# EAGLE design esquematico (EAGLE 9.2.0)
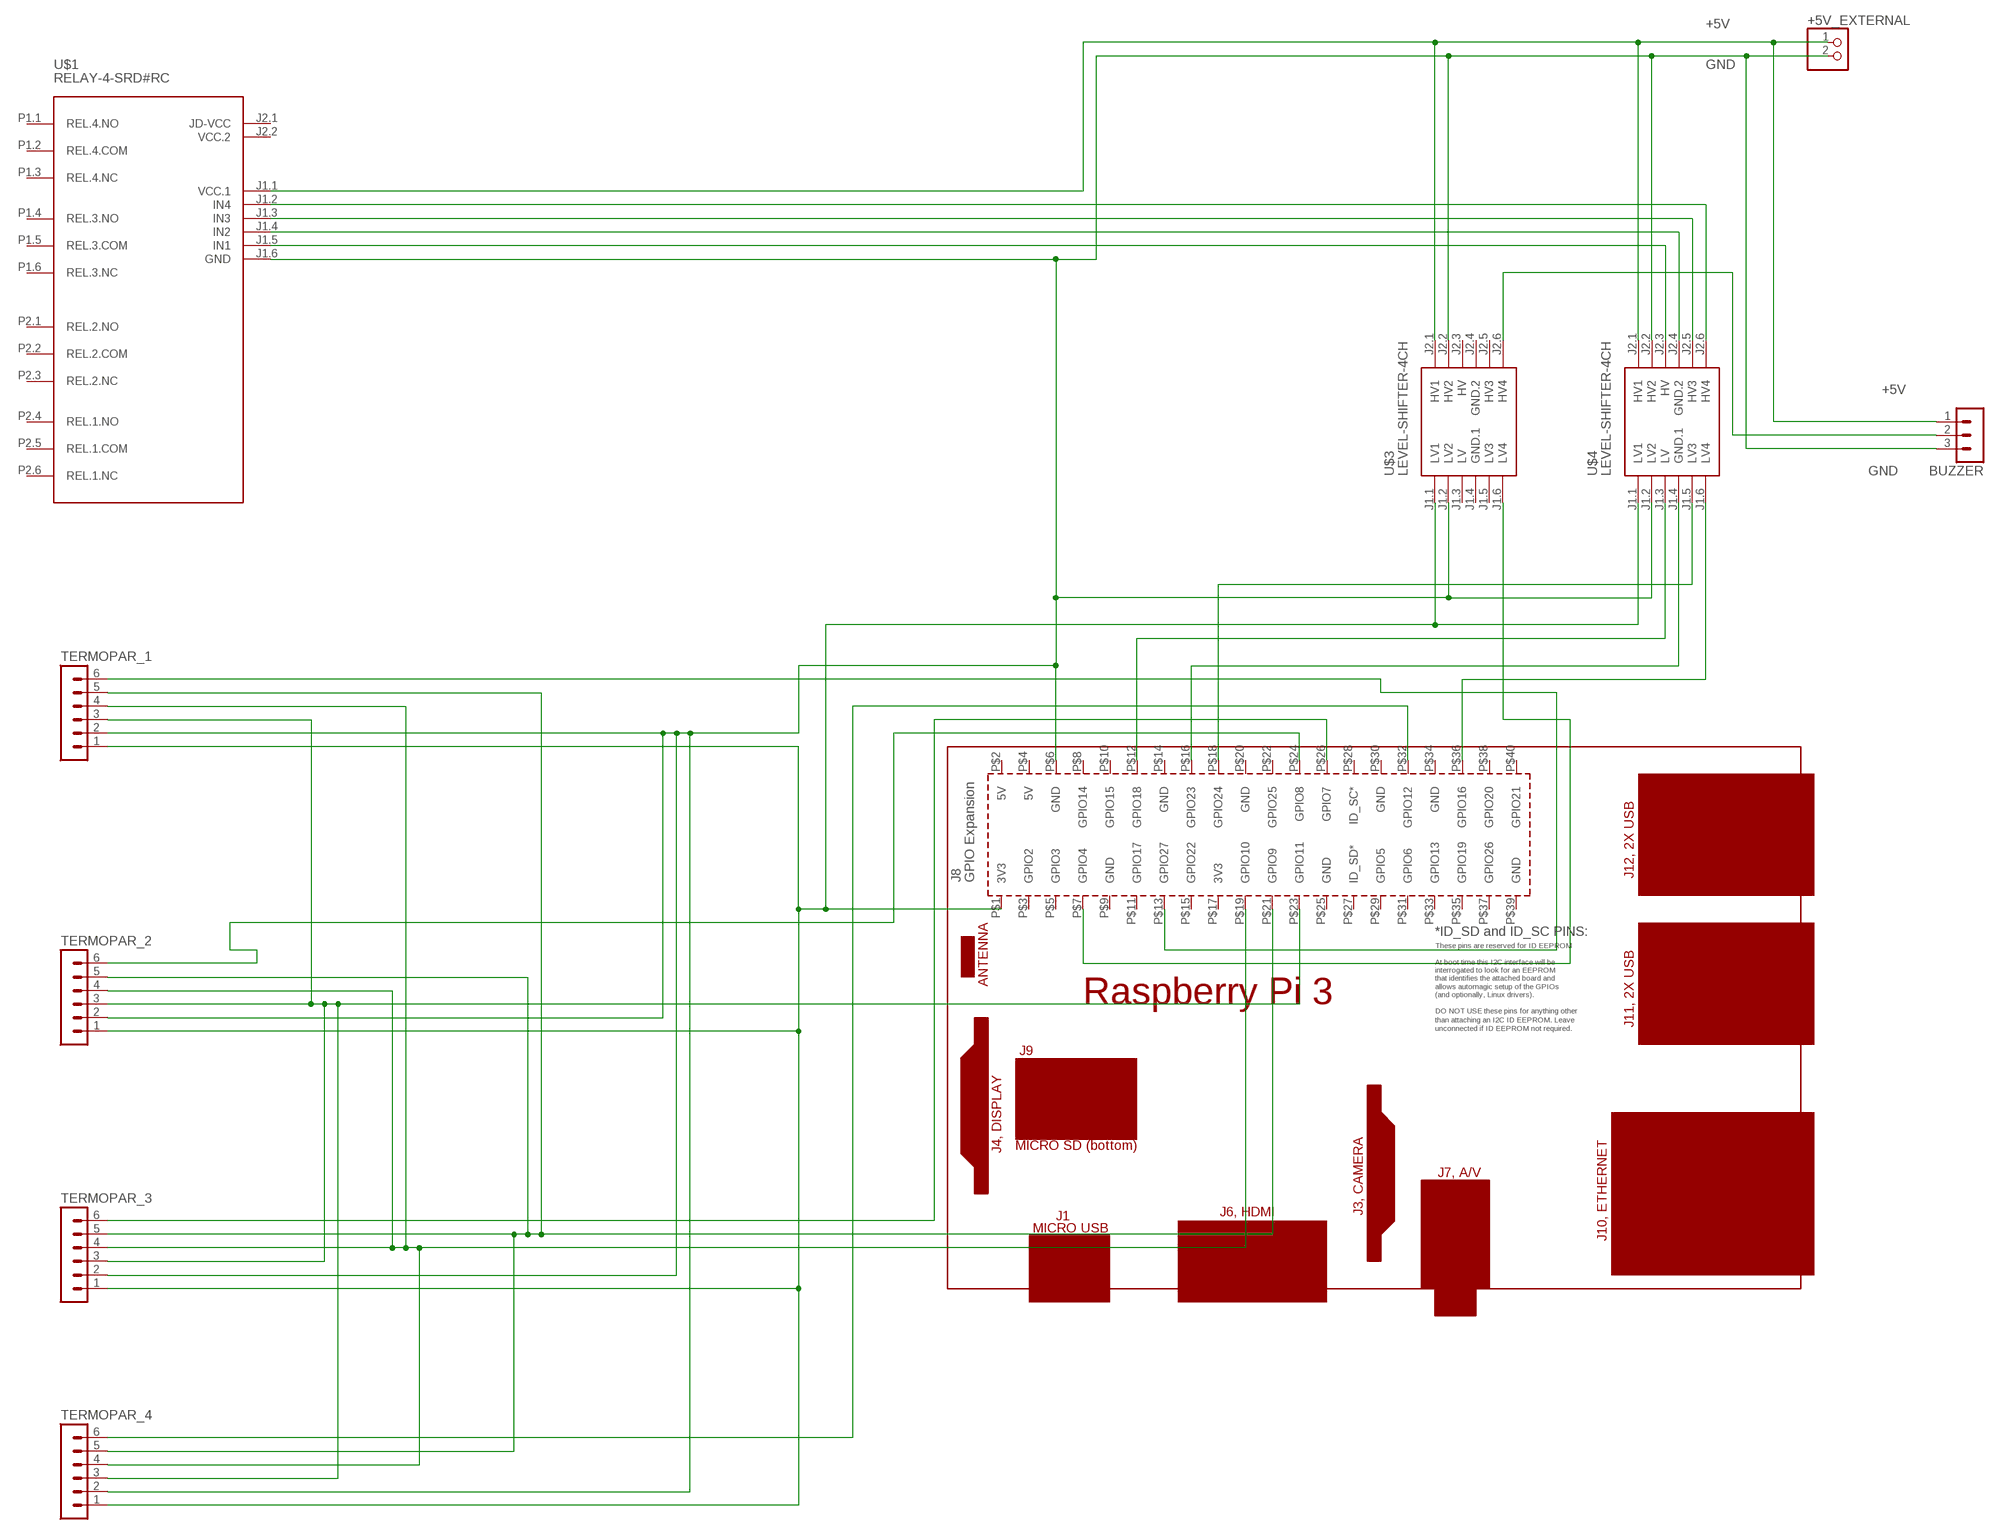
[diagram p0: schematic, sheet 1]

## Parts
+5V_EXTERNAL  PINHD-1X2  [1X02]
BUZZER  MA03-1  [MA03-1]
PCB1  RPI3RPI3  [RPI3]
TERMOPAR_1  MA06-1  [MA06-1]
TERMOPAR_2  MA06-1  [MA06-1]
TERMOPAR_3  MA06-1  [MA06-1]
TERMOPAR_4  MA06-1  [MA06-1]
U$1  RELAY-4-SRD#RC  [RELAY-4-SRD#RC]
U$3  LEVEL-SHIFTER-4CH  [LEVEL-SHIFTER-4CH]
U$4  LEVEL-SHIFTER-4CH  [LEVEL-SHIFTER-4CH]

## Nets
+5V: +5V_EXTERNAL.1 BUZZER.1 U$1.J1.1(VCC.1) U$3.J2.1(HV1) U$4.J2.1(HV1)
GND: +5V_EXTERNAL.2 BUZZER.3 PCB1.P$6(GND) TERMOPAR_1.2 TERMOPAR_2.2 TERMOPAR_3.2 TERMOPAR_4.2 U$1.J1.6(GND) U$3.J1.2(LV2) U$3.J2.2(HV2) U$4.J1.2(LV2) U$4.J2.2(HV2)
N$1: U$1.J1.2(IN4) U$4.J2.6(HV4)
N$2: U$1.J1.3(IN3) U$4.J2.5(HV3)
N$3: U$1.J1.4(IN2) U$4.J2.4(GND.2)
N$4: U$1.J1.5(IN1) U$4.J2.3(HV)
N$5: PCB1.P$12(GPIO18) U$4.J1.3(LV)
N$6: PCB1.P$16(GPIO23) U$4.J1.4(GND.1)
N$7: PCB1.P$18(GPIO24) U$4.J1.5(LV3)
N$8: PCB1.P$36(GPIO16) U$4.J1.6(LV4)
N$9: PCB1.P$7(GPIO4) U$3.J1.6(LV4)
N$10: BUZZER.2 U$3.J2.6(HV4)
N$14: PCB1.P$1(3V3) TERMOPAR_1.1 TERMOPAR_2.1 TERMOPAR_3.1 TERMOPAR_4.1 U$3.J1.1(LV1) U$4.J1.1(LV1)
N$16: PCB1.P$23(GPIO11) TERMOPAR_1.3 TERMOPAR_2.3 TERMOPAR_3.3 TERMOPAR_4.3
N$17: PCB1.P$19(GPIO10) TERMOPAR_1.4 TERMOPAR_2.4 TERMOPAR_3.4 TERMOPAR_4.4
N$18: PCB1.P$21(GPIO9) TERMOPAR_1.5 TERMOPAR_2.5 TERMOPAR_3.5 TERMOPAR_4.5
N$19: PCB1.P$13(GPIO27) TERMOPAR_1.6
N$21: PCB1.P$26(GPIO7) TERMOPAR_3.6
N$22: PCB1.P$32(GPIO12) TERMOPAR_4.6
S$20: PCB1.P$24(GPIO8) TERMOPAR_2.6
Unconnected: PCB1.P$2(5V) PCB1.P$3(GPIO2) PCB1.P$4(5V) PCB1.P$5(GPIO3) PCB1.P$8(GPIO14) PCB1.P$9(GND) PCB1.P$10(GPIO15) PCB1.P$11(GPIO17) PCB1.P$14(GND) PCB1.P$15(GPIO22) PCB1.P$17(3V3) PCB1.P$20(GND) PCB1.P$22(GPIO25) PCB1.P$25(GND) PCB1.P$27(ID_SD*) PCB1.P$28(ID_SC*) PCB1.P$29(GPIO5) PCB1.P$30(GND) PCB1.P$31(GPIO6) PCB1.P$33(GPIO13) PCB1.P$34(GND) PCB1.P$35(GPIO19) PCB1.P$37(GPIO26) PCB1.P$38(GPIO20) PCB1.P$39(GND) PCB1.P$40(GPIO21) U$1.J2.1(JD-VCC) U$1.P1.1(REL.4.NO) U$1.P1.2(REL.4.COM) U$1.P1.3(REL.4.NC) U$1.P1.4(REL.3.NO) U$1.P1.5(REL.3.COM) U$1.P1.6(REL.3.NC) U$1.P2.1(REL.2.NO) U$1.P2.2(REL.2.COM) U$1.P2.3(REL.2.NC) U$1.P2.4(REL.1.NO) U$1.P2.5(REL.1.COM) U$1.P2.6(REL.1.NC) U$3.J1.5(LV3) U$3.J2.5(HV3)

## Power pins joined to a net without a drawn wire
GND.1: U$3.J1.4(GND.1)
GND.2: U$3.J2.4(GND.2)
HV: U$3.J2.3(HV)
LV: U$3.J1.3(LV)
VCC.2: U$1.J2.2(VCC.2)

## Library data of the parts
+5V_EXTERNAL = pinhead:PINHD-1X2: PIN HEADER
BUZZER = con-lstb:MA03-1: PIN HEADER; OC_FARNELL: unknown; OC_NEWARK: unknown
PCB1 = e14_Rpi3_RevA+mirror-pcb:RPI3: Device for Raspberry Pi 3 board created by Dave Young for www.element14.com More information and support community is available at https://www.element14.com/community/community/raspberry-pi Device for Raspberry Pi 3 board updated by Gerald Schwarz for www.element14.com On RPI3 addet the layer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
TERMOPAR_1-TERMOPAR_4 = con-lstb:MA06-1: PIN HEADER; OC_FARNELL: unknown; OC_NEWARK: unknown
U$1 = diy-modules:RELAY-4-SRD#RC: 4-Channel Relay Module based on SRD-05VDC-SL-C relays Symbol with relays pins Click here to find device on ebay.com
U$3 U$4 = diy-modules_modified:LEVEL-SHIFTER-4CH: 4-Channel Bi-Directional Logic Level Converter based on BSS128 transistors Click here to find device on ebay.com

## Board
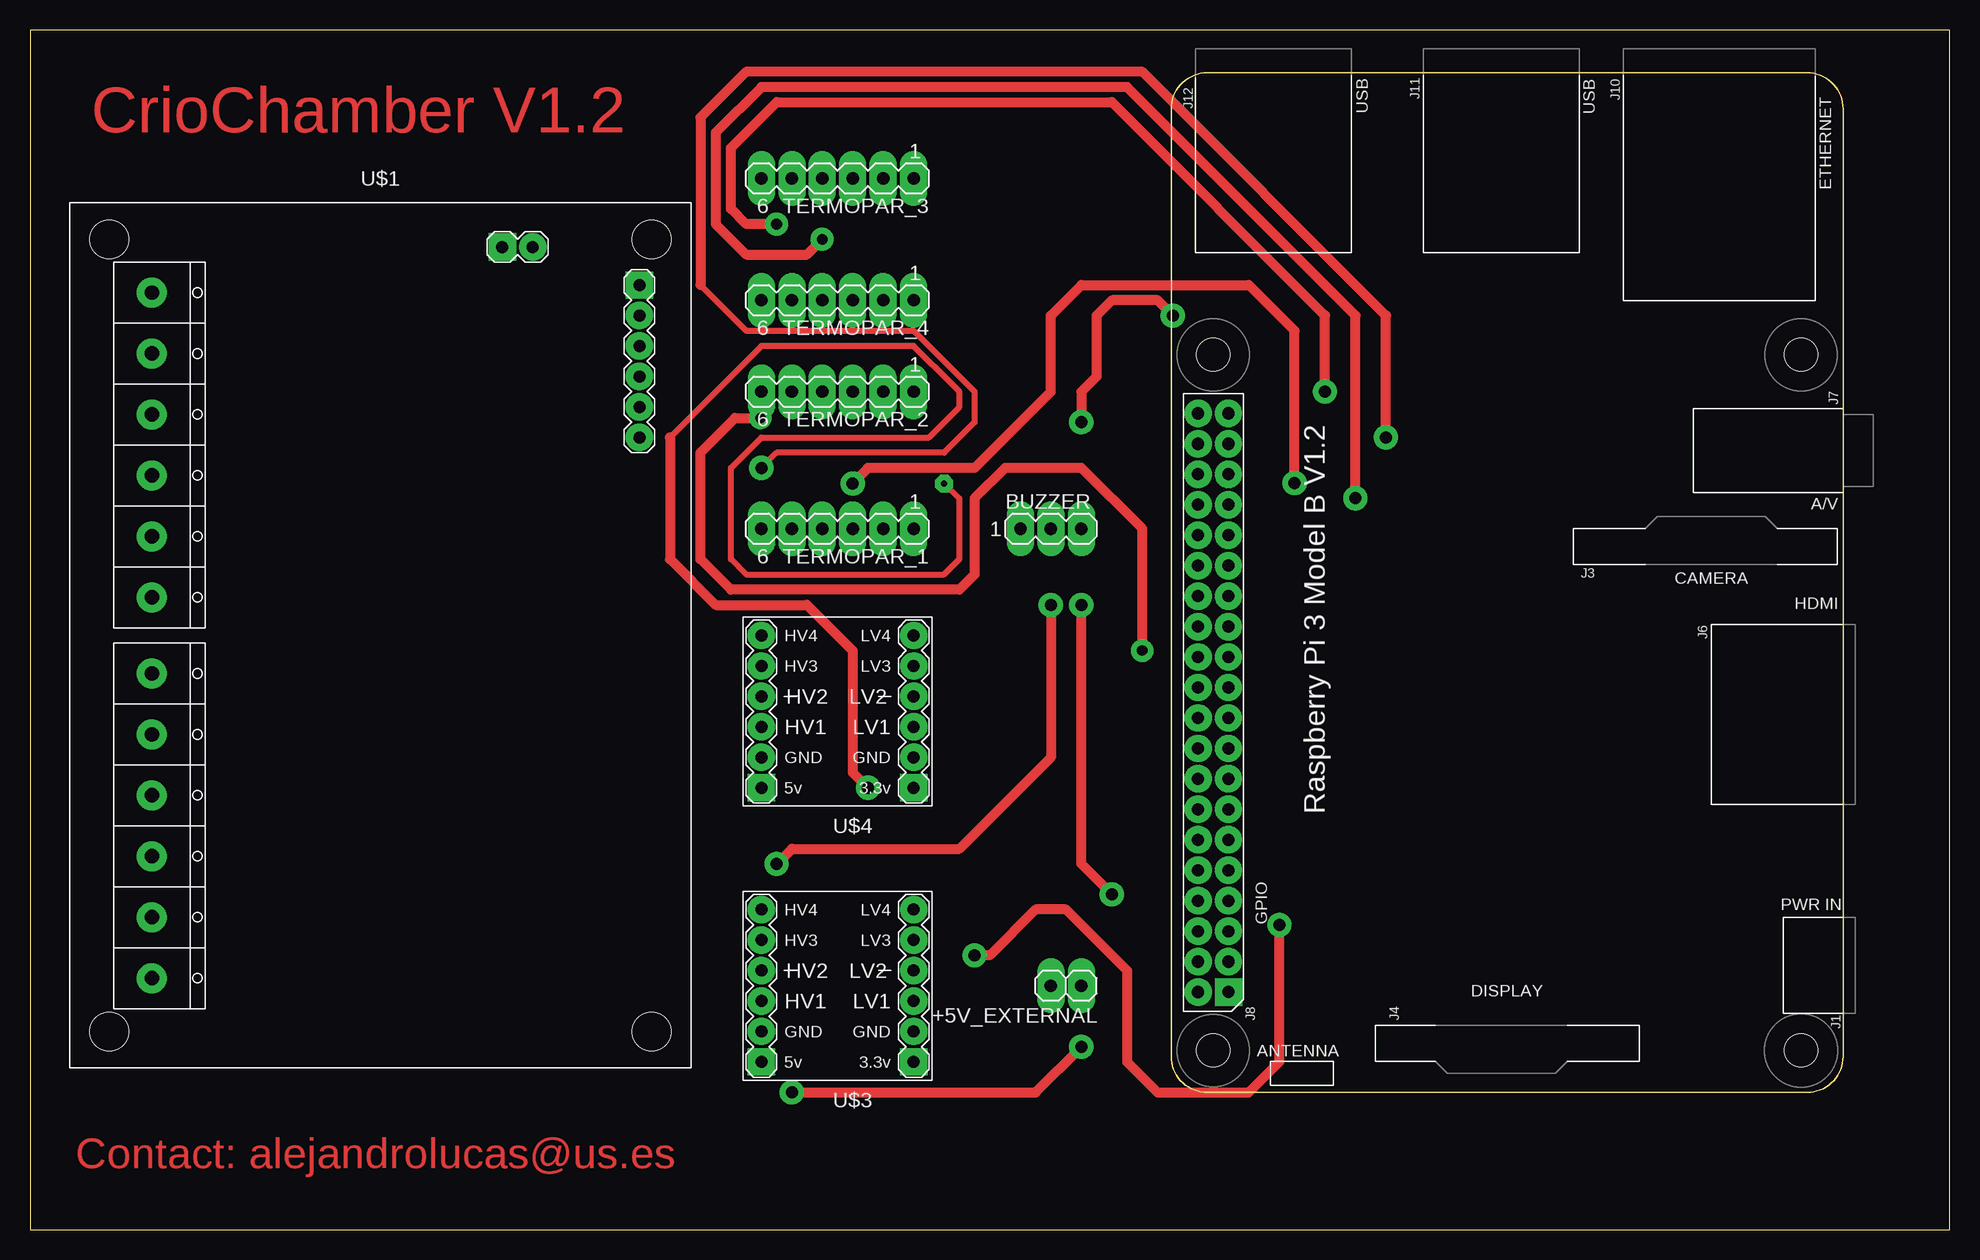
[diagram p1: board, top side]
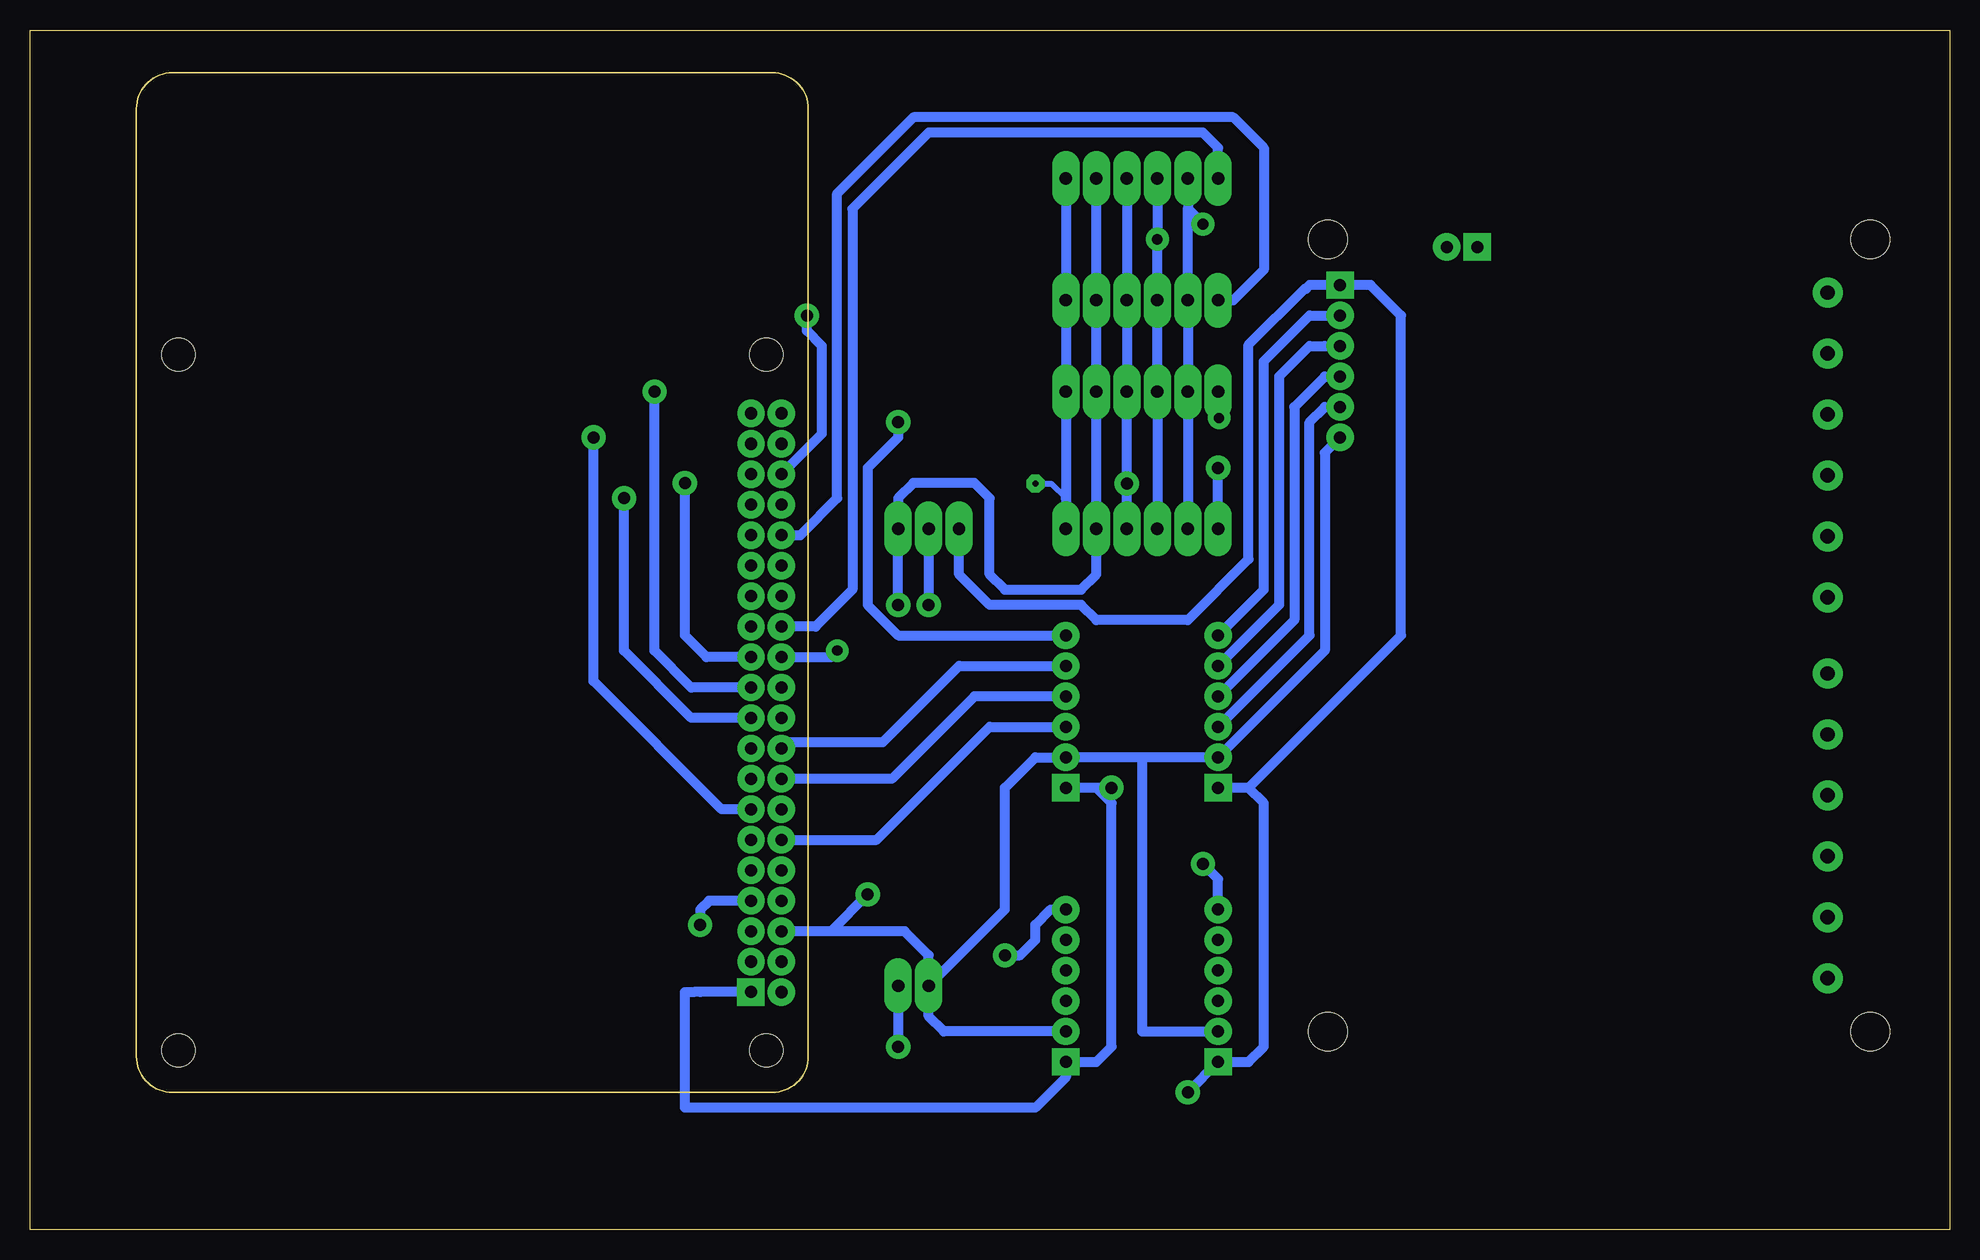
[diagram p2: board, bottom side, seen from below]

Size 160 x 100 mm. Coordinates in mm from the lower left corner, seen from the top.
Outline: 0,0 160,0 160,100 0,100 0,0
Copper layers (1*16): Top 0.035mm / dielectric 1.5mm / Bottom 0.035mm
Design rules "default *": minimum track width 6mil, minimum drill 0.35mm, track to track 6mil, track to pad 6mil, pad to pad 6mil, via to via 6mil, smd to smd 6mil, copper to edge 40mil, drill to drill 6mil, minimum pad ring 25mil, minimum via ring 20mil, stop-mask expansion 4mil, vias tented up to drill 0mil, thermal gap 10mil

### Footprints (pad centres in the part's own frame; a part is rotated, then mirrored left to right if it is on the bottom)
1X02 = drill 1.016 long: 1 -1.27,0; 2 1.27,0
MA03-1 = drill 1.016 long: 1 -2.54,0; 2 0,0; 3 2.54,0
RPI3 = drill 1.016 square: P$1 8.37,51.23 | drill 1.016: P$2 8.357,53.772; P$3 10.897,51.232; P$4 10.897,53.772; P$5 13.437,51.232; P$6 13.437,53.772; P$7 15.977,51.232; P$8 15.977,53.772; P$9 18.517,51.232; P$10 18.517,53.772; P$11 21.057,51.232; P$12 21.057,53.772; P$13 23.597,51.232; P$14 23.597,53.772; P$15 26.137,51.232; P$16 26.137,53.772; P$17 28.677,51.232; P$18 28.677,53.772; P$19 31.217,51.232; P$20 31.217,53.772; P$21 33.757,51.232; P$22 33.757,53.772; P$23 36.297,51.232; P$24 36.297,53.772; P$25 38.837,51.232; P$26 38.837,53.772; P$27 41.377,51.232; P$28 41.377,53.772; P$29 43.917,51.232; P$30 43.917,53.772; P$31 46.457,51.232; P$32 46.457,53.772; P$33 48.997,51.232; P$34 48.997,53.772; P$35 51.537,51.232; P$36 51.537,53.772; P$37 54.077,51.232; P$38 54.077,53.772; P$39 56.617,51.232; P$40 56.617,53.772 | hole 2.75: 3.5,3.5; 61.5,3.5; 3.5,52.5; 61.5,52.5
MA06-1 = drill 1.016 long: 1 -6.35,0; 2 -3.81,0; 3 -1.27,0; 4 1.27,0; 5 3.81,0; 6 6.35,0
RELAY-4-SRD#RC = drill 1 square: J1.1 20.32,29.21; J2.1 8.89,32.385 | drill 1: J1.2 20.32,26.67; J1.3 20.32,24.13; J1.4 20.32,21.59; J1.5 20.32,19.05; J1.6 20.32,16.51; J2.2 11.43,32.385 | drill 1.2 pad 2.5: P1.1 -20.32,28.575; P1.2 -20.32,23.495; P1.3 -20.32,18.415; P1.4 -20.32,13.335; P1.5 -20.32,8.255; P1.6 -20.32,3.175; P2.1 -20.32,-3.175; P2.2 -20.32,-8.255; P2.3 -20.32,-13.335; P2.4 -20.32,-18.415; P2.5 -20.32,-23.495; P2.6 -20.32,-28.575 | hole 3.2: -23.876,33.02; 21.336,33.02; 21.336,-33.02; -23.876,-33.02
LEVEL-SHIFTER-4CH = drill 1 square: J1.1 -5.08,6.35; J2.1 7.62,6.35 | drill 1: J1.2 -5.08,3.81; J1.3 -5.08,1.27; J1.4 -5.08,-1.27; J1.5 -5.08,-3.81; J1.6 -5.08,-6.35; J2.2 7.62,3.81; J2.3 7.62,1.27; J2.4 7.62,-1.27; J2.5 7.62,-3.81; J2.6 7.62,-6.35

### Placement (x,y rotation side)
+5V_EXTERNAL  86.36,20.32 180 top
BUZZER  85.09,58.42 0 top
PCB1  151.13,11.43 90 top
TERMOPAR_1  67.31,58.42 180 top
TERMOPAR_2  67.31,69.85 180 top
TERMOPAR_3  67.31,87.63 180 top
TERMOPAR_4  67.31,77.47 180 top
U$1  30.48,49.53 0 top
U$3  68.58,20.32 180 top
U$4  68.58,43.18 180 top

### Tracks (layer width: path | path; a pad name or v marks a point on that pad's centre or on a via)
+5V  (via drill 1)
  Top 0.813: v87.63,15.24 83.82,11.43 v63.5,11.43
  Bottom 0.813: 58.42,36.83 45.72,49.53 45.72,76.2 48.26,78.74 U$1.J1.1 53.34,78.74 53.65,78.44 53.74,78.44 58.42,73.75 58.42,55.88 63.5,50.8 71.12,50.8 72.39,52.07 80.01,52.07 82.55,54.61 BUZZER.1 | 58.42,36.83 57.15,35.56 57.15,15.24 58.42,13.97 U$3.J2.1 v63.5,11.43 | +5V_EXTERNAL.1 v87.63,15.24 | 58.42,36.83 U$4.J2.1
GND  (via drill 1)
  Top 0.813: v90.17,27.94 87.63,30.48 v87.63,52.07
  Bottom 0.813: 67.31,39.37 U$4.J2.2 52.07,48.26 52.07,64.77 U$1.J1.6 | 67.31,39.37 U$4.J1.2 76.2,39.37 78.74,36.83 78.74,26.67 +5V_EXTERNAL.2 | U$3.J2.2 67.31,16.51 67.31,39.37 | TERMOPAR_3.2 TERMOPAR_4.2 TERMOPAR_2.2 TERMOPAR_1.2 71.12,54.61 72.39,53.34 78.74,53.34 80.01,54.61 80.01,60.96 81.28,62.23 86.36,62.23 87.63,60.96 BUZZER.3 v87.63,52.07 | +5V_EXTERNAL.2 85.09,22.86 87.1,24.87 93.24,24.87 | 93.24,24.87 PCB1.P$6 | +5V_EXTERNAL.2 85.09,17.78 83.82,16.51 U$3.J1.2 | v90.17,27.94 93.24,24.87
N$1
  Bottom 0.813: U$1.J1.2 53.34,76.2 57.15,72.39 57.15,53.34 U$4.J2.6
N$2
  Bottom 0.813: U$4.J2.5 55.88,52.07 55.88,71.12 53.34,73.66 52.07,73.66 U$1.J1.3
N$3
  Bottom 0.813: U$4.J2.4 54.61,50.8 54.61,68.58 52.07,71.12 U$1.J1.4
N$4
  Bottom 0.813: U$4.J2.3 53.34,49.53 53.34,67.31 52.07,68.58 U$1.J1.5
N$5
  Bottom 0.813: PCB1.P$12 89.43,32.49 80.01,41.91 U$4.J1.3
N$6
  Bottom 0.813: PCB1.P$16 88.16,37.57 81.28,44.45 U$4.J1.4
N$7
  Bottom 0.813: PCB1.P$18 96.83,40.64 88.9,40.64 82.55,46.99 U$4.J1.5
N$8  (via drill 1)
  Top 0.813: v87.63,67.31 87.63,69.85 88.9,71.12 88.9,76.2 90.17,77.47 93.98,77.47 v95.25,76.2
  Bottom 0.813: v87.63,67.31 87.63,66.04 90.17,63.5 90.17,52.07 87.63,49.53 U$4.J1.6 | PCB1.P$36 93.98,66.34 93.98,73.66 95.25,74.93 v95.25,76.2
N$9  (via drill 1)
  Top 0.813: v104.14,25.4 104.14,13.97 101.6,11.43 93.98,11.43 91.44,13.97 91.44,21.59 86.36,26.67 83.82,26.67 80.01,22.86 v78.74,22.86
  Bottom 0.813: PCB1.P$7 103.4,27.41 104.14,26.67 v104.14,25.4 | v78.74,22.86 77.47,22.86 76.2,24.13 76.2,25.4 74.93,26.67 U$3.J1.6
N$10  (via drill 1)
  Top 0.813: v85.09,52.07 85.09,39.37 77.47,31.75 63.5,31.75 v62.23,30.48
  Bottom 0.813: BUZZER.2 v85.09,52.07 | U$3.J2.6 60.96,29.21 v62.23,30.48
N$14  (via drill 0.5 pad 1.3, 1)
  Top 0.508: 53.34,66.04 60.96,73.66 73.66,73.66 76.83,70.48 77.47,69.85 77.47,68.58 74.93,66.04 60.96,66.04 58.42,63.5 58.42,55.88 59.69,54.61 76.2,54.61 77.47,55.88 77.47,60.96 77.42,60.96 v76.2,62.18
  Top 0.813: 53.34,66.04 53.34,55.88 57.15,52.07 64.77,52.07 68.58,48.26 68.58,38.1 v69.85,36.83
  Bottom 0.508: v76.2,62.18 74.88,62.18 73.66,60.96
  Bottom 0.813: TERMOPAR_3.1 TERMOPAR_4.1 TERMOPAR_2.1 73.66,60.96 TERMOPAR_1.1 | PCB1.P$1 104.14,19.8 104.66,19.8 105.41,19.8 105.41,10.16 76.2,10.16 73.66,12.7 U$3.J1.1 71.12,13.97 69.85,15.24 69.85,35.56 71.12,36.83 U$4.J1.1 v69.85,36.83
N$16  (via drill 1)
  Top 0.813: v105.41,62.23 105.41,74.93 101.6,78.74 87.63,78.74 85.09,76.2 85.09,69.85 78.74,63.5 69.85,63.5 68.58,62.23 v68.58,62.19
  Bottom 0.813: TERMOPAR_3.3 TERMOPAR_4.3 TERMOPAR_2.3 v68.58,62.19 TERMOPAR_1.3 | PCB1.P$23 103.61,47.73 105.41,49.53 v105.41,62.23
N$17  (via drill 0.9, 1)
  Top 0.813: v110.49,60.96 110.49,76.2 91.44,95.25 60.96,95.25 57.15,91.44 57.15,83.82 59.69,81.28 64.77,81.28 v66.04,82.55
  Bottom 0.813: TERMOPAR_1.4 TERMOPAR_2.4 TERMOPAR_4.4 | 66.04,78.74 TERMOPAR_4.4 | TERMOPAR_3.4 v66.04,82.55 TERMOPAR_4.4 | PCB1.P$19 104.88,42.65 110.49,48.26 v110.49,60.96
N$18  (via drill 0.9, 1)
  Top 0.813: v107.95,69.85 107.95,76.2 90.17,93.98 62.23,93.98 58.42,90.17 58.42,85.09 59.69,83.82 v62.23,83.82
  Bottom 0.813: TERMOPAR_1.5 TERMOPAR_2.5 TERMOPAR_4.5 63.5,85.09 | PCB1.P$21 104.88,45.19 107.95,48.26 v107.95,69.85 | TERMOPAR_3.5 63.5,85.09 | 63.5,85.09 v62.23,83.82
N$19  (via drill 1)
  Top 0.508: 55.88,78.74 59.69,74.93 73.66,74.93 78.74,69.85 78.74,67.31 76.2,64.77 62.23,64.77 v60.96,63.5
  Top 0.813: 55.88,78.74 55.88,92.71 59.69,96.52 92.71,96.52 113.03,76.2 v113.03,66.04
  Bottom 0.813: PCB1.P$13 102.34,35.03 113.03,45.72 v113.03,66.04 | TERMOPAR_1.6 v60.96,63.5
N$21
  Bottom 0.813: TERMOPAR_3.6 60.96,90.17 62.23,91.44 85.09,91.44 91.44,85.09 91.44,53.34 94.51,50.27 PCB1.P$26
N$22
  Bottom 0.813: PCB1.P$32 95.78,57.89 92.71,60.96 92.71,86.36 86.36,92.71 59.69,92.71 57.15,90.17 57.15,80.01 59.69,77.47 TERMOPAR_4.6
S$20  (via drill 0.85)
  Top 0.813: v92.71,48.26 92.71,58.42 87.63,63.5 81.28,63.5 78.74,60.96 78.74,54.61 77.47,53.34 58.42,53.34 55.88,55.88 55.88,64.77 58.77,67.66 v60.89,67.66
  Bottom 0.813: PCB1.P$24 93.24,47.73 v92.71,48.26 | v60.89,67.66 60.96,67.73 TERMOPAR_2.6

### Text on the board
Top: CrioChamber V1.2 | Contact: alejandrolucas@us.es

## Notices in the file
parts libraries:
diy-modules: Released under the Creative Commons Attribution 4.0 International License: http://creativecommons.org/licenses/by/4.0
